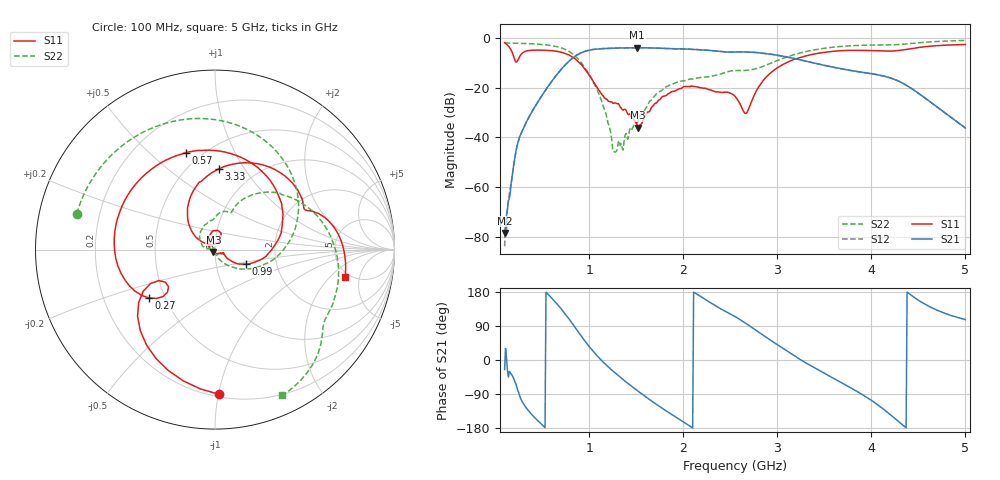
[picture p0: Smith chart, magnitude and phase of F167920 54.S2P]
!  2-Port S-parameters saved by WinCal
! VAR MeasName=S-Parameters (CALIBRATED_DATA) read from VNA (N5242A)
! VAR MeasDate=2016-11-22 9:58:10
! VAR NAME=F167920 54
! VAR FILENAME=F167920 54.S2P
! VAR DATE=2016-11-22 9:58:10
! VAR PHYS_PORTS=1,2
# Hz S DB R 50
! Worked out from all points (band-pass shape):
!   491 points, 100 MHz to 5 GHz, reference 50 ohm
!   highest |S21| = -3.88 dB at 1.51 GHz (marker M1); lowest = -78.4 dB at 100 MHz (marker M2)
!   |S21| within 3 dB of the highest: 867.6 MHz to 2.994 GHz (2.126 GHz wide, 110 % of centre)
!   lowest |S11| = -36.1 dB at 1.52 GHz (marker M3), VSWR 1.03, Z = 49.1 - j1.28 ohm
!   |S11| at or under -10 dB: 896.2 MHz to 3.092 GHz (2.195 GHz wide, 110 % of centre)
!   |S22| runs from -45.9 to -1.0 dB; largest |S21 - S12| = 0.0012
!   S11 on the Smith chart (normalised r, x): 100 MHz: 0.22, -1.01; 270 MHz: 0.41, -0.28; 570 MHz: 0.42, +0.66; 990 MHz: 1.39, -0.23; 3.33 GHz: 0.69, +0.77; 5 GHz: 4.56, -3.09
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1e8  -1.86 -88.2  -78.45 -25.4  -83.76 39.0  -1.98 165.5
1.6e8  -4.23 -132.6  -62.23 -33.2  -60.45 -34.7  -2.02 156.7
2e8  -7.83 -152.2  -50.25 -50.9  -50.09 -53.4  -2.05 150.8
2.7e8  -6.83 -143.7  -38.86 -101.0  -38.90 -100.4  -2.13 140.2
3.9e8  -4.90 165.9  -29.71 -144.4  -29.69 -144.2  -2.31 120.8
5.7e8  -4.97 106.6  -19.06 171.6  -19.06 171.6  -2.88 86.6
7.6e8  -6.43 45.0  -10.22 116.5  -10.22 116.5  -4.86 37.8
9.2e8  -10.83 -7.3  -5.82 61.8  -5.82 61.8  -10.14 -13.0
9.9e8  -14.40 -25.0  -4.97 38.4  -4.97 38.4  -14.03 -33.1
1.16e9  -23.97 -31.2  -4.20 -8.5  -4.20 -8.5  -28.61 -71.9
1.27e9  -26.11 -20.7  -4.08 -33.2  -4.08 -33.2  -45.91 -145.0
1.51e9  -35.02 -115.8  -3.88 -80.5  -3.88 -80.5  -34.13 164.9
1.52e9  -36.10 -123.8  -3.90 -82.5  -3.90 -82.5  -33.22 171.5
1.74e9  -24.89 133.4  -4.09 -121.3  -4.08 -121.3  -21.74 156.4
2.11e9  -19.45 80.2  -4.55 179.1  -4.55 179.2  -16.38 107.8
2.55e9  -23.40 61.2  -5.63 114.8  -5.63 114.7  -13.09 73.0
2.67e9  -30.24 108.8  -5.60 95.8  -5.59 95.8  -13.02 66.8
2.91e9  -14.66 138.6  -6.39 55.3  -6.39 55.2  -10.45 62.7
3.33e9  -6.94 87.3  -9.53 -11.4  -9.54 -11.5  -5.22 28.3
3.37e9  -6.58 83.0  -9.87 -17.2  -9.88 -17.3  -4.91 24.6
4.19e9  -5.25 24.3  -15.88 -141.8  -15.91 -141.7  -2.77 -32.4
5e9  -2.60 -11.9  -36.24 106.6  -36.12 107.3  -0.97 -65.2
